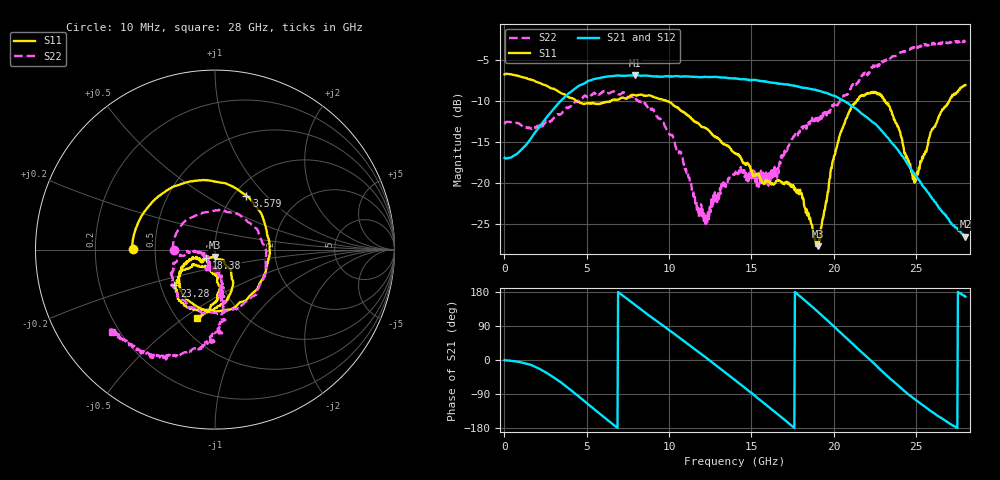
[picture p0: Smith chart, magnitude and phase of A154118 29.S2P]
!  2-Port S-parameters saved by WinCal
! VAR MeasName=S-Parameters (CALIBRATED_DATA) read from VNA (N5230A)
! VAR MeasDate=2015-9-10 14:36:34
! VAR NAME=A154118 29
! VAR FILENAME=A154118 29.S2P
! VAR DATE=2015-9-10 14:36:34
! VAR PHYS_PORTS=1,2
# Hz S DB R 50
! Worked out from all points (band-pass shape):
!   801 points, 10 MHz to 28 GHz, reference 50 ohm
!   highest |S21| = -6.89 dB at 7.952 GHz (marker M1); lowest = -26.5 dB at 28 GHz (marker M2)
!   |S21| within 3 dB of the highest: 3.485 GHz to 20.5 GHz (17.02 GHz wide, 142 % of centre)
!   lowest |S11| = -27.7 dB at 19.04 GHz (marker M3), VSWR 1.09, Z = 49.7 - j4.11 ohm
!   |S11| at or under -10 dB: 4.368 GHz to 6.475 GHz (2.107 GHz wide, 38.9 % of centre); 9.824 GHz to 21.43 GHz (11.6 GHz wide, 74.3 % of centre); 23.12 GHz to 27.02 GHz (3.901 GHz wide, 15.6 % of centre)
!   |S22| runs from -25.3 to -2.7 dB; largest |S21 - S12| = 0.0078
!   S11 on the Smith chart (normalised r, x): 10 MHz: 0.37, +0.00; 3.579 GHz: 1.14, +0.78; 18.38 GHz: 0.90, -0.09; 23.28 GHz: 0.59, -0.26; 28 GHz: 0.62, -0.56
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1e7  -6.79 179.6  -16.94 -0.2  -17.02 -0.1  -12.84 180.0
1.9693e9  -7.71 117.5  -13.59 -20.2  -13.60 -19.9  -13.23 86.1
3.578725e9  -9.19 59.7  -9.71 -64.0  -9.70 -64.2  -11.25 5.0
4.698325e9  -10.32 18.6  -8.04 -102.9  -8.02 -103.2  -9.78 -41.7
6.377725e9  -10.09 -35.8  -7.02 -162.4  -6.99 -162.5  -9.05 -94.6
7.952162e9  -9.35 -79.6  -6.89 144.7  -6.86 144.7  -9.63 -129.7
9.351662e9  -9.74 -112.3  -7.08 99.3  -7.01 99.2  -12.06 -159.1
1.06462e10  -11.06 -134.9  -7.04 58.0  -6.97 57.7  -16.23 -175.9
1.218565e10  -13.31 -150.2  -7.08 8.3  -7.05 7.7  -24.07 -127.4
1.4005e10  -16.38 -158.4  -7.30 -53.0  -7.30 -53.6  -18.91 -113.2
1.578936e10  -20.04 -149.9  -7.62 -114.7  -7.60 -115.0  -18.72 -95.5
1.715388e10  -19.85 -137.7  -8.00 -162.9  -7.97 -163.3  -16.09 -76.1
1.837844e10  -23.42 -135.9  -8.47 152.5  -8.46 152.0  -12.99 -80.5
1.869332e10  -25.16 -122.8  -8.59 140.6  -8.64 140.1  -12.06 -81.3
1.90432e10  -27.69 -92.0  -8.78 126.8  -8.71 126.4  -12.50 -81.4
1.995288e10  -17.23 -51.3  -9.37 91.2  -9.35 90.5  -10.70 -80.1
2.10025e10  -11.18 -75.0  -10.51 48.5  -10.48 47.8  -8.57 -83.7
2.327669e10  -10.40 -138.6  -14.48 -42.9  -14.49 -44.0  -5.09 -99.8
2.334666e10  -10.64 -138.2  -14.62 -45.9  -14.64 -46.7  -5.01 -100.8
2.495609e10  -19.29 -113.3  -19.06 -104.4  -19.09 -104.5  -3.61 -116.1
2.649554e10  -11.46 -87.5  -23.27 -152.2  -23.25 -152.5  -2.93 -130.2
2.8e10  -8.08 -104.5  -26.55 167.4  -26.46 167.4  -2.66 -141.2
